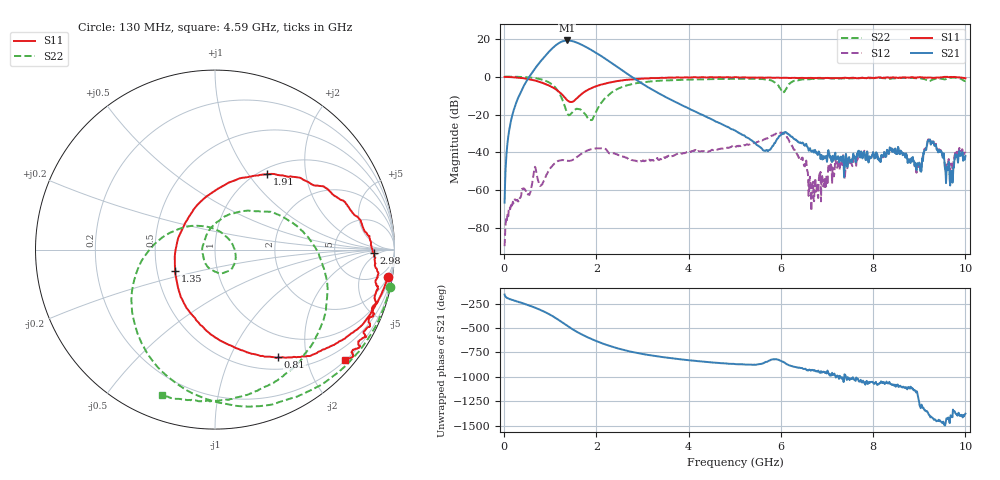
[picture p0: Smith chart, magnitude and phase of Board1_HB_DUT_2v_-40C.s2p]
! Created Tue May 27 11:35:58 2025
# hz S ma R 50
! 2 Port Network Data from SP1.SP block
! freq  magS11  angS11  magS21  angS21  magS12  angS12  magS22  angS22
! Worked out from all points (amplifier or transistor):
!   1000 points, 10 MHz to 10 GHz, reference 50 ohm
!   highest |S21| = 19.1 dB at 1.36 GHz (marker M1)
!   |S21| within 3 dB of that: 1.097 GHz to 1.739 GHz (642 MHz wide, 45.3 % of centre)
!   unconditionally stable (mu >= 1): 19.55 MHz to 23.12 MHz; 86.78 MHz to 109.4 MHz; 110.6 MHz to end of sweep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
!   at 1.67 GHz: K = 6.80, MAG = 17.6 dB, |S12| = -40.8 dB
!   at 5.01 GHz: K = 11.38, MAG = -9.3 dB, |S12| = -37.1 dB
!   at 10 GHz: K = 405.21, MAG = -30.2 dB, |S12| = -39.6 dB
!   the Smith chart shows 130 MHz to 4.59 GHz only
!   S11 on the Smith chart (normalised r, x): 130 MHz: 2, -12; 810 MHz: 0.66, -1.54; 1.35 GHz: 0.62, -0.16; 1.91 GHz: 1.09, +1.24; 2.98 GHz: 16, -3; 4.59 GHz: 0.20, -2.71
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1e7  0.9817 -1.0  0.0004733 -157.6  3.347e-05 150.4  1.005 -0.8
1.3e8  0.9745 -9.1  0.05345 155.2  0.0003152 72.9  0.9984 -12.0
5.6e8  0.8441 -39.3  1.062 88.0  0.0008495 113.0  0.9477 -55.9
8.1e8  0.6955 -59.6  2.723 39.9  0.00139 95.2  0.8449 -90.5
9.7e8  0.5819 -74.8  4.515 2.9  0.003399 117.6  0.7083 -119.8
1.12e9  0.4652 -94.0  6.731 -38.4  0.005434 99.5  0.4999 -156.2
1.25e9  0.3443 -120.3  8.435 -79.3  0.006215 81.6  0.2676 159.5
1.35e9  0.2502 -152.2  9.004 -111.8  0.00607 73.6  0.1229 99.3
1.36e9  0.2428 -156.8  9.032 -115.1  0.006049 73.3  0.1146 90.9
1.51e9  0.2264 133.3  8.471 -160.6  0.006593 76.7  0.1269 -25.9
1.68e9  0.3478 85.0  6.956 154.8  0.009308 71.0  0.1263 -85.8
1.91e9  0.5111 55.2  4.911 104.0  0.01233 46.8  0.0724 148.9
2.24e9  0.6766 31.7  2.706 44.4  0.01067 2.9  0.3066 44.4
2.55e9  0.7927 15.1  1.498 0.0  0.007944 -1.3  0.529 6.4
2.98e9  0.8849 -1.3  0.6688 -43.8  0.005865 10.5  0.705 -28.9
3.34e9  0.92 -12.4  0.3685 -71.2  0.006416 12.9  0.7755 -51.2
4.59e9  0.9533 -40.4  0.06489 -135.0  0.01198 1.6  0.8651 -110.1
5.01e9  0.9721 -48.1  0.03759 -149.3  0.01402 -8.5  0.8753 -126.5
6.05e9  0.9321 -69.2  0.03239 -125.0  0.03292 -100.9  0.3745 -155.4
6.67e9  0.9227 -87.4  0.01039 151.8  0.000928 -134.0  0.8761 -156.3
8.34e9  0.9408 -134.2  0.009165 14.6  0.009053 8.8  0.8678 164.1
1e10  0.9093 -164.1  0.008079 63.6  0.01045 62.7  0.7782 128.4
